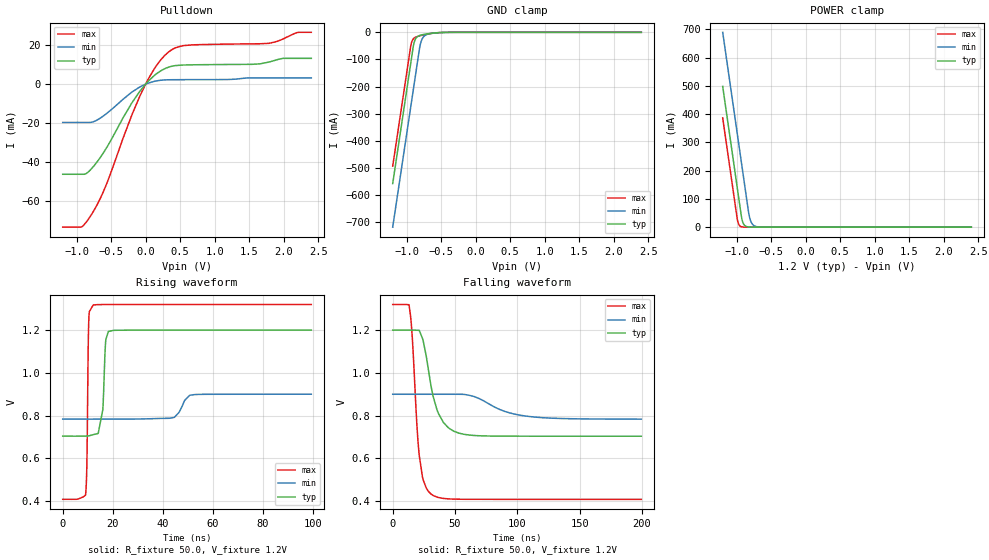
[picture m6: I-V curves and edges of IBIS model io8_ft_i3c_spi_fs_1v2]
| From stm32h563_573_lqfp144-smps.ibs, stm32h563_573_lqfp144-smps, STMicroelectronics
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[Model]   io8_ft_i3c_spi_fs_1v2
Model_type I/O_open_drain
Polarity   Non-Inverting
Enable   Active-Low
| CAP_THRESHOLD on pad IOFT is "UDTCAPC" :
| Rising=20.0% of vddiom   Falling=80.0% of vddiom
| C_comp min and max val. don't necessarily correlate with the min and max pvt
| but are the smallest and greatest pad capacitance found.
| var   typ   min   max
C_comp   3.41735pF  3.39645pF  3.42910pF
|C_comp_pulldown   3.41735pF  3.39645pF  3.42910pF
Vinl = 450.0mV
Vinh = 660.0mV
Vmeas = 600.0mV   | Reference voltage for timing measurements
Cref  = 50.0pF   | Timing specification test load capacitance value
Rref  = 1.0MOhm   | Timing specification test load resistance value
Vref  = 660.0mV   | Timing specification test load voltage
[Model Spec]
| TIME_THRESHOLD on pin ZII2CV11 is "CMOS" :
| Rising=40.0% of vdd   Falling=60.0% of vdd
Vinl 447.80000mV 344.80000mV 489.80000mV
Vinh 733.20000mV 535.20000mV 813.20000mV
| variable   typ   min   max
[Temperature Range] 25.0 125.0 -40.0
| variable   typ   min   max
[Voltage Range] 1.2V 900.0mV 1.32V
| variable   typ   min   max
[POWER Clamp Reference] 1.2V 900.0mV 1.32V
| variable   typ   min   max
[GND Clamp Reference] 0V 0V 0V
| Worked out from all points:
|   slope of the pulldown table from 0 to 0.18 V, typ, clamps not added: 30.6 ohm
|   GND clamp passes 1 mA (typ) near -0.52 V on its own axis
|   POWER clamp passes 1 mA (typ) near -0.84 V on its own axis
|   rising waveform, R_fixture 50.0, V_fixture 1.2V: 20-80 % time 1.32ns typ, 3.38ns min, 534ps max; typ from 0.704 V to 1.2 V
|   falling waveform, R_fixture 50.0, V_fixture 1.2V: 20-80 % time 11.2ns typ, 27.5ns min, 5.88ns max; typ from 1.2 V to 0.704 V
[POWER Clamp]
-1.2V     497.8mA    689.2mA    386.5mA
-990mV    140.8mA    332.2mA    29.53mA
-980mV    123.8mA    315.2mA    17.95mA
-960mV    89.81mA    281.2mA    6.634mA
-930mV    38.81mA    230.2mA    1.49mA
-900mV    12.07mA    179.2mA    334.8uA
-870mV    3.756mA    128.2mA    75.22uA
-820mV    536.4uA    44.98mA    6.246uA
-790mV    166.9uA    18.76mA    1.403uA
-750mV    35.18uA    5.846mA    191.8nA
-590mV    70.09nA    55uA       165.5pA
2.4V      0A         0A         0A
[GND Clamp]
-1.2V     -558.2mA   -719mA     -494.1mA
-940mV    -116.2mA   -277mA     -52.06mA
-930mV    -99.19mA   -260mA     -39.94mA
-900mV    -49.1mA    -209mA     -23.76mA
-880mV    -30.14mA   -175mA     -19.6mA
-850mV    -17.82mA   -124mA     -16.09mA
-810mV    -11.73mA   -56.78mA   -12.91mA
-780mV    -9.444mA   -28.21mA   -10.92mA
-740mV    -7.291mA   -13.16mA   -8.574mA
-640mV    -3.573mA   -4.171mA   -3.954mA
-380mV    -61.75uA   -230.3uA   -20.32uA
2.4V      3.863nA    718.4nA    150.6pA
| variable   typ   min   max
[Pullup Reference] 1.2V 900.0mV 1.32V
| variable   typ   min   max
[Pulldown Reference] 0V 0V 0V
[Pulldown]
-1.2V     -46.17mA   -19.62mA   -73.27mA
-930mV    -46.17mA   -19.62mA   -73.18mA
-770mV    -42.8mA    -19.41mA   -66.04mA
-570mV    -32.88mA   -15.18mA   -51.58mA
-200mV    -9.658mA   -4.083mA   -15.89mA
-80mV     -3.488mA   -1.363mA   -5.887mA
120mV     4.232mA    1.387mA    7.501mA
340mV     8.782mA    2.251mA    16.66mA
540mV     9.805mA    2.305mA    19.74mA
1.79V     11.33mA    3.206mA    20.93mA
2.2V      13.23mA    3.206mA    26.48mA
2.4V      13.23mA    3.206mA    26.56mA
[Ramp]
dV/dt_r 297.79741mV/1.02832ns 69.90053mV/3.0598ns 547.13371mV/532.48965ps
dV/dt_f 297.80506mV/10.97931ns 69.86866mV/27.34375ns 547.13935mV/5.7267ns
R_load = 50.0
| Removed startup time: 0s 0s 0s  .
| Removed end time: 99.4ns.
[Rising Waveform]
R_fixture   = 50.0
V_fixture   = 1.2V
V_fixture_min = 900.0mV
V_fixture_max = 1.32V
0s        703.7mV    783.5mV    408.1mV
9.15ns    704mV      783.5mV    431mV
9.65ns    704.4mV    783.5mV    566.8mV
10.2ns    705.1mV    783.5mV    1.122V
10.45ns   705.5mV    783.5mV    1.252V
12.2ns    710.7mV    783.5mV    1.318V
16.05ns   828.7mV    783.5mV    1.32V
17.15ns   1.143V     783.5mV    1.32V
18.25ns   1.193V     783.5mV    1.32V
99.4ns    1.2V       900mV      1.32V
| Removed startup time: 0s 0s 0s  .
| Removed end time: 199.4ns.
[Falling Waveform]
R_fixture   = 50.0
V_fixture   = 1.2V
V_fixture_min = 900.0mV
V_fixture_max = 1.32V
0s        1.2V       900mV      1.32V
13.1ns    1.2V       900mV      1.317V
15.45ns   1.2V       900mV      1.187V
21.3ns    1.199V     900mV      612.7mV
24.5ns    1.149V     900mV      498mV
31.2ns    924.6mV    900mV      431mV
40.7ns    767.6mV    900mV      412.3mV
57ns      712.7mV    899.5mV    408.3mV
105.8ns   703.7mV    798.6mV    408.1mV
199.4ns   703.7mV    783.6mV    408.1mV
